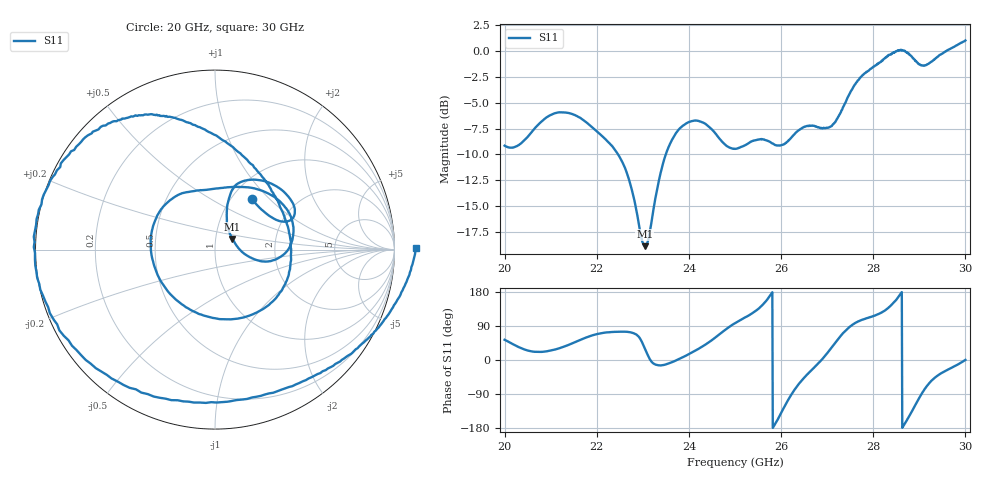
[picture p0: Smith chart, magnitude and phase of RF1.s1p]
! freq	mag(S11)	phase(S11)
!ADF5904 RF1
#  Hz  S  MA  R 50
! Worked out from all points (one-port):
!   1001 points, 20 GHz to 30 GHz, reference 50 ohm
!   lowest |S11| = -18.9 dB at 23.04 GHz (marker M1), VSWR 1.26, Z = 60.3 + j7.26 ohm
!   |S11| at or under -10 dB: 22.46 GHz to 23.5 GHz (1.036 GHz wide, 4.51 % of centre)
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2e10  0.3485 53.3
2.063e10  0.4162 21.9
2.125e10  0.5051 33.6
2.18e10  0.4469 60.7
2.25e10  0.3062 74.6
2.304e10  0.1141 31.4
2.341e10  0.2706 -14.1
2.375e10  0.4092 0.4
2.424e10  0.4562 31.7
2.5e10  0.3368 97.3
2.548e10  0.3722 132.5
2.58e10  0.3581 176.9
2.599e10  0.3497 -142.3
2.625e10  0.3883 -86.1
2.655e10  0.4332 -40.2
2.687e10  0.4241 -1.0
2.717e10  0.4526 44.4
2.75e10  0.6294 88.6
2.797e10  0.8256 114.5
2.83e10  0.9385 135.0
2.845e10  0.9774 151.9
2.857e10  1.008 170.3
2.875e10  0.9729 -154.7
2.887e10  0.9208 -128.8
2.898e10  0.8647 -103.9
2.93e10  0.8986 -50.5
2.959e10  0.9986 -27.3
3e10  1.122 0.3
